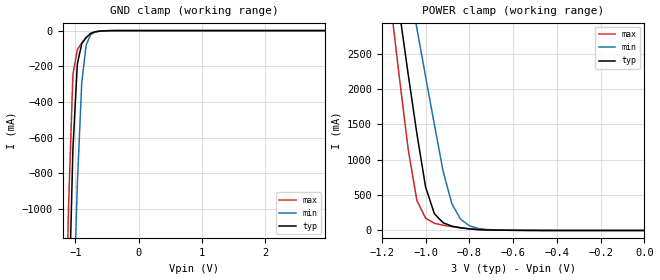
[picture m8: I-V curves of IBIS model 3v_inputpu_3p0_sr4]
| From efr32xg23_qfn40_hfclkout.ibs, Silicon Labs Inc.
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|   Model 3v_inputpu_3p0_sr4
[Model]  3v_inputpu_3p0_sr4
Model_type Input
C_comp   1.6300pF   1.4000pF   2.7000pF
[Temperature Range]   25.0000   0.1250k   -40.0000
[Pullup Reference]   3.0000V   2.7000V   3.3000V
[Pulldown Reference]   0.0V   0.0V   0.0V
[POWER Clamp Reference]   3.0000V   2.7000V   3.3000V
[GND Clamp Reference]   0.0V   0.0V   0.0V
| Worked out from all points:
|   GND clamp passes 1 mA (typ) near -0.51 V on its own axis
|   POWER clamp passes 1 mA (typ) near -0.53 V on its own axis
[GND_clamp]
|Voltage   I(typ)   I(min)   I(max)
-3V       -32.58A    -30.59A    -34.3A
-1.18V    -2.82A     -3.643A    -2.261A
-1.11V    -1.645A    -2.575A    -1.001A
-1.04V    -666.5mA   -1.673A    -246.6mA
-970mV    -186.8mA   -861.8mA   -106.8mA
-900mV    -73.94mA   -290.7mA   -69.08mA
-830mV    -38.09mA   -80.54mA   -39.72mA
-760mV    -16.05mA   -23.08mA   -17.46mA
-690mV    -6.69mA    -7.915mA   -7.391mA
-410mV    -193.6uA   -358uA     -153.4uA
2.95V     -1.126uA   11.14uA    -9.136uA
[POWER_clamp]
|Voltage   I(typ)   I(min)   I(max)
-3V       48.87A     43.6A      53.88A
-1.16V    4.025A     5.101A     3.218A
-1.12V    3.102A     4.315A     2.168A
-1.08V    2.218A     3.569A     1.158A
-1.04V    1.373A     2.862A     425.9mA
-1V       614.2mA    2.175A     173.2mA
-960mV    237.5mA    1.499A     101.5mA
-920mV    109mA      838.4mA    74.92mA
-880mV    61.27mA    377.2mA    54.04mA
-840mV    37.85mA    159.1mA    37.07mA
-720mV    7.423mA    13.59mA    7.883mA
0V        1.008nA    10.52nA    1.016nA
